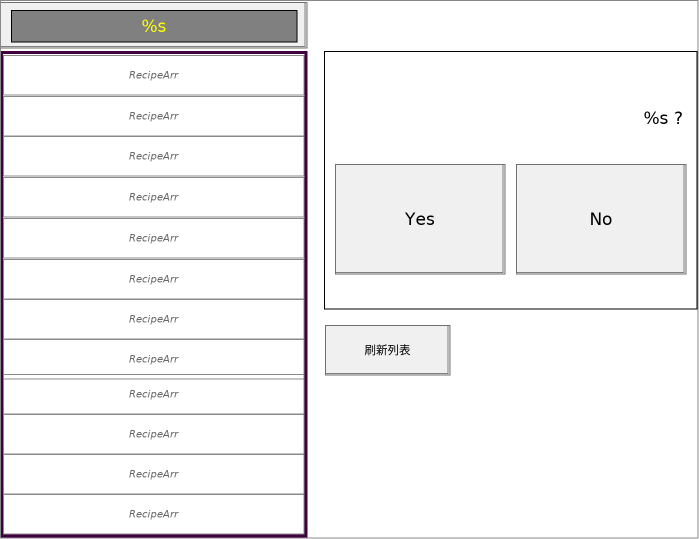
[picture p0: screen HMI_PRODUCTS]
VISUALIZATION HMI_PRODUCTS  // 699x539
    Rectangle (0,51 307x486)
    Button (-1,2 308x46)
    Rectangle (11,10 286x32), "%s", text variable: .strCurrentReceipeName
    Rectangle (325,145 125x58), "输入配方名"
    Button (325,55 126x68), "读取"
        tap vbtLoad
    Button (460,55 118x68), "保存"
        tap vbtSave
    Button (590,55 100x68), "删除"
        tap vbtdel
    Rectangle (450,145 243x58), "%s", text variable: strInputReceipeName
        OnMouseDown: write the text variable via Default
    Button (325,230 126x68), "从USB读取"
        tap vbtLoadFromUSB
    Button (460,230 118x68), "下载到USB"
        tap vbtSaveToUSB
    Button (325,325 125x50), "刷新列表", pressed state: .vbtFlash
        toggle .vbtFlash
    Group (324,51 373x258), invisible if: NOT ShowDiag
        Rectangle (0,0 373x258), invisible if: (NOT .ShowDiag) <> 0
        Rectangle (129,35 244x64), "%s ?", text variable: strShowDiagName
        Button (11,113 170x110), "Yes"
            tap vbtYes
        Button (192,113 170x110), "No"
            tap vbtNo
        Rectangle (13,35 209x64), text list: 'question', text index: DiagIndex
    Frame (3,55 301x40)
        shows RecipeArr(ID := 1)
    Frame (3,96 301x40)
        shows RecipeArr(ID := 2)
    Frame (3,136 301x40)
        shows RecipeArr(ID := 3)
    Frame (3,177 301x40)
        shows RecipeArr(ID := 4)
    Frame (3,218 301x40)
        shows RecipeArr(ID := 5)
    Frame (3,259 301x40)
        shows RecipeArr(ID := 6)
    Frame (3,299 301x40)
        shows RecipeArr(ID := 7)
    Frame (3,339 301x40)
        shows RecipeArr(ID := 8)
    Frame (3,374 301x40)
        shows RecipeArr(ID := 9)
    Frame (3,414 301x40)
        shows RecipeArr(ID := 10)
    Frame (3,454 301x40)
        shows RecipeArr(ID := 11)
    Frame (3,494 301x40)
        shows RecipeArr(ID := 12)
END_VISUALIZATION
